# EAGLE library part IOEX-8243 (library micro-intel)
MICROCOMPUTER/PERIPHERAL DEVICE
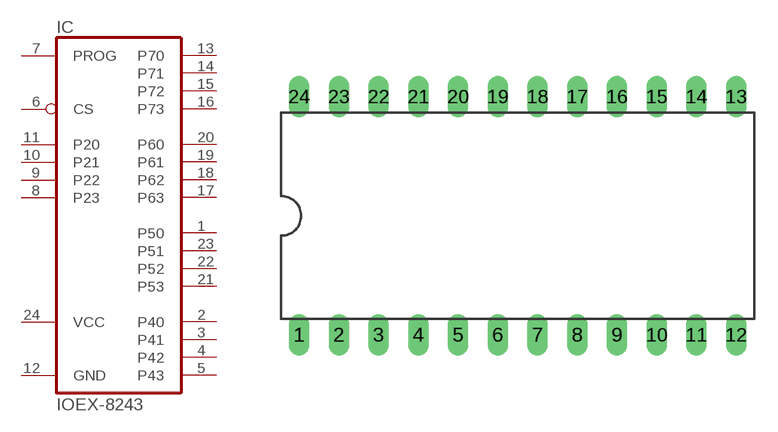
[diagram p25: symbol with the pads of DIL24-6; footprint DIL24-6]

Designator prefix IC

## IOEX-8243 (OC_FARNELL: unknown; OC_NEWARK: unknown)  [DIL24-6]
1  P50
2  P40
3  P41
4  P42
5  P43
6  CS  in
7  PROG  in
8  P23
9  P22
10  P21
11  P20
12  GND  pwr
13  P70
14  P71
15  P72
16  P73
17  P63
18  P62
19  P61
20  P60
21  P53
22  P52
23  P51
24  VCC  pwr

## Footprint DIL24-6 (pad centres in mm)
Dual In Line Package 0.6 inch
drill 0.813 long: 1 -13.97,-7.62; 2 -11.43,-7.62; 3 -8.89,-7.62; 4 -6.35,-7.62; 5 -3.81,-7.62; 6 -1.27,-7.62; 7 1.27,-7.62; 8 3.81,-7.62; 9 6.35,-7.62; 10 8.89,-7.62; 11 11.43,-7.62; 12 13.97,-7.62; 13 13.97,7.62; 14 11.43,7.62; 15 8.89,7.62; 16 6.35,7.62; 17 3.81,7.62; 18 1.27,7.62; 19 -1.27,7.62; 20 -3.81,7.62; 21 -6.35,7.62; 22 -8.89,7.62; 23 -11.43,7.62; 24 -13.97,7.62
